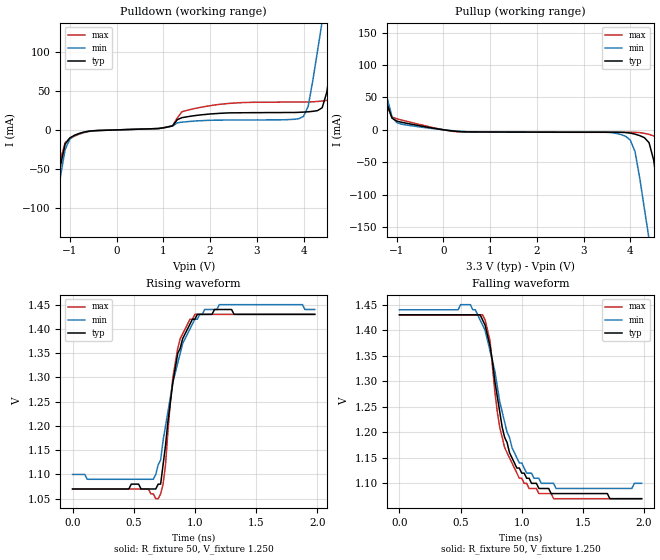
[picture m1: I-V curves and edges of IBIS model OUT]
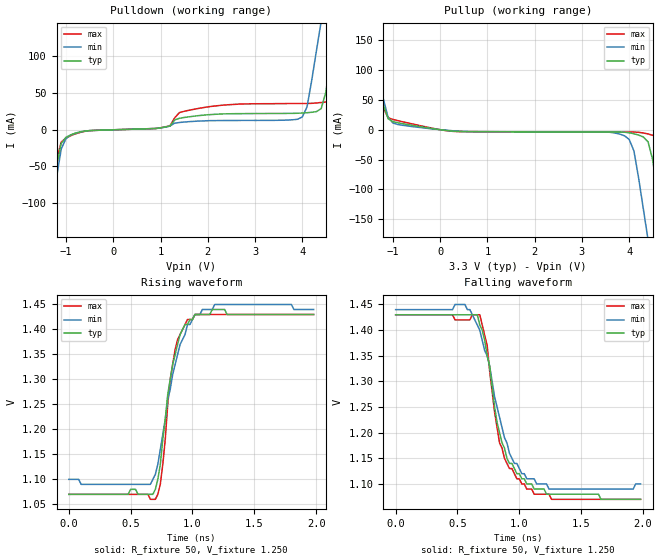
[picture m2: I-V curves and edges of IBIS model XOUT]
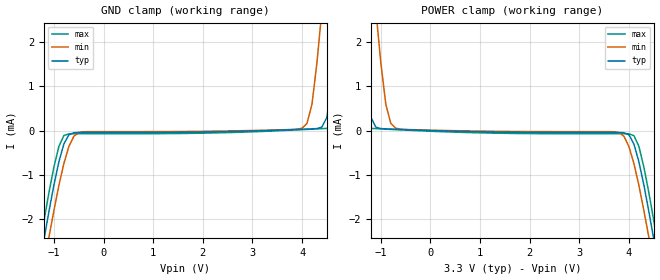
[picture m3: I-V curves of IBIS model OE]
| IBIS File sg5032van_33v.ibs
[IBIS Ver] 3.2
[File name] sg5032van_33v.ibs
[File Rev] 1
[Date] May 1 2013
[Source]
[Disclaimer]
Seiko Epson Corporation makes no warranty with respect to the information
contained herein.
[Copyright]
Copyright(C) 2013 Seiko Epson Corporation. All rights reserved.
| Component SG5032VAN 3.3V
[Component] sg5032van_33v
[Manufacturer] Seiko Epson Corporation
[Package]
R_pkg 0.046 NA NA
L_pkg 0.61n NA NA
C_pkg 0.95p NA NA
[Pin] signal_name model_name R_pin L_pin C_pin
1 OE OE
2 GND GND
3 GND GND
4 OUT OUT 0.046 0.61n 0.95p
5 XOUT XOUT 0.046 0.61n 0.95p
6 VCC POWER
[Diff Pin] inv_pin vdiff tdelay_typ
4 5 0 0
| Models and submodels in the file (3): OUT (Output), XOUT (Output), OE (Input)
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[Model] OUT
Model_type Output
Enable Active-High
Polarity Non-Inverting
Vref=1.250
Vmeas=1.250
Rref=50
Cref=0
C_comp 0.12p 0.12p 0.12p
[Temperature Range] 25 105 -40
[Voltage Range] 3.3 2.97 3.63
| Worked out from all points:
|   slope of the pulldown table from 0 to 0.495 V, typ, clamps not added: 507 ohm
|   slope of the pullup table from 0 to 0.495 V, typ, clamps not added: 153 ohm
|   falling waveform, R_fixture 50, V_fixture 1.250: 20-80 % time 188ps typ, 196ps min, 167ps max; typ from 1.43 V to 1.07 V
|   rising waveform, R_fixture 50, V_fixture 1.250: 20-80 % time 125ps typ, 165ps min, 92.4ps max; typ from 1.07 V to 1.43 V
[Pullup]
-3.3V     961mA      849mA      1.08A
-1.5V     170mA      162mA      181mA
-1.2V     39mA       48.2mA     34.7mA
-900mV    11.8mA     8.83mA     15.3mA
3.9V      -4.13mA    -10mA      -3.85mA
4.1V      -6.66mA    -33.8mA    -3.9mA
4.4V      -19.9mA    -169mA     -7.09mA
4.6V      -99.3mA    -264mA     -12.4mA
4.7V      -153mA     -312mA     -16.5mA
4.8V      -207mA     -360mA     -30.1mA
5.1V      -369mA     -503mA     -198mA
6.6V      -1.18A     -1.22A     -1.1A
[Pulldown]
-3.3V     -1.19A     -1.07A     -1.31A
-1.4V     -152mA     -155mA     -154mA
-1.2V     -45.9mA    -59.6mA    -38.1mA
-1.1V     -18.2mA    -25.2mA    -16.5mA
-900mV    -6.98mA    -7.24mA    -8.05mA
3.9V      22.4mA     14.3mA     35.6mA
4.1V      23.1mA     30mA       35.7mA
4.4V      28.3mA     139mA      36.9mA
4.7V      135mA      253mA      39.9mA
4.8V      179mA      291mA      46.7mA
5V        266mA      366mA      133mA
6.6V      969mA      975mA      937mA
[Falling Waveform]
R_fixture=50
V_fixture=1.250
V_fixture_min=1.271
V_fixture_max=1.238
0s        1.43V      1.44V      1.43V
580ps     1.43V      1.45V      1.43V
680ps     1.42V      1.41V      1.43V
740ps     1.37V      1.36V      1.38V
800ps     1.27V      1.29V      1.24V
860ps     1.19V      1.22V      1.17V
960ps     1.13V      1.15V      1.12V
1.06ns    1.11V      1.12V      1.09V
1.28ns    1.08V      1.09V      1.07V
1.98ns    1.07V      1.1V       1.07V
[Rising Waveform]
R_fixture=50
V_fixture=1.250
V_fixture_min=1.271
V_fixture_max=1.238
0s        1.07V      1.1V       1.07V
660ps     1.07V      1.09V      1.06V
700ps     1.08V      1.12V      1.05V
720ps     1.08V      1.13V      1.06V
740ps     1.12V      1.17V      1.08V
820ps     1.29V      1.29V      1.3V
860ps     1.35V      1.33V      1.36V
1ns       1.42V      1.42V      1.43V
1.2ns     1.44V      1.45V      1.43V
1.98ns    1.43V      1.44V      1.43V
[Ramp]
R_load=50
dV/dt_r 2.133E-1/1.209E-10 2.089E-1/1.701E-10 2.153E-1/9.119E-11
dV/dt_f 2.130E-1/1.860E-10 2.090E-1/2.110E-10 2.147E-1/1.643E-10
|[End OUT
[Model] XOUT
Model_type Output
Enable Active-High
Polarity Inverting
Vref=1.250
Vmeas=1.250
Rref=50
Cref=0
C_comp 0.12p 0.12p 0.12p
[Temperature Range] 25 105 -40
[Voltage Range] 3.3 2.97 3.63
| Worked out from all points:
|   slope of the pulldown table from 0 to 0.495 V, typ, clamps not added: 506 ohm
|   slope of the pullup table from 0 to 0.495 V, typ, clamps not added: 153 ohm
|   falling waveform, R_fixture 50, V_fixture 1.250: 20-80 % time 181ps typ, 204ps min, 151ps max; typ from 1.43 V to 1.07 V
|   rising waveform, R_fixture 50, V_fixture 1.250: 20-80 % time 123ps typ, 159ps min, 93.9ps max; typ from 1.07 V to 1.43 V
[Pullup]
-3.3V     1.03A      904mA      1.18A
-1.5V     183mA      173mA      197mA
-1.2V     41.5mA     51.3mA     36.6mA
-900mV    11.8mA     8.85mA     15.4mA
3.9V      -4.13mA    -10.1mA    -3.85mA
4.1V      -6.68mA    -35.4mA    -3.9mA
4.4V      -20.3mA    -185mA     -7.11mA
4.6V      -110mA     -289mA     -12.4mA
4.7V      -169mA     -341mA     -16.7mA
4.8V      -229mA     -393mA     -31.5mA
5.1V      -408mA     -549mA     -221mA
6.6V      -1.3A      -1.33A     -1.24A
[Pulldown]
-3.3V     -1.32A     -1.17A     -1.48A
-1.4V     -168mA     -170mA     -172mA
-1.2V     -49.6mA    -64.8mA    -40.9mA
-1.1V     -18.6mA    -26.1mA    -16.8mA
-900mV    -7.02mA    -7.27mA    -8.11mA
3.9V      22.5mA     14.3mA     35.7mA
4.1V      23.2mA     31.1mA     35.8mA
4.4V      28.8mA     148mA      37.1mA
4.7V      145mA      269mA      40.2mA
4.8V      192mA      309mA      48.2mA
5V        286mA      390mA      145mA
6.6V      1.04A      1.04A      1.02A
[Falling Waveform]
R_fixture=50
V_fixture=1.250
V_fixture_min=1.271
V_fixture_max=1.238
0s        1.43V      1.44V      1.43V
560ps     1.43V      1.45V      1.42V
660ps     1.43V      1.41V      1.43V
680ps     1.41V      1.4V       1.43V
740ps     1.35V      1.35V      1.37V
840ps     1.2V       1.23V      1.18V
920ps     1.14V      1.16V      1.13V
1.06ns    1.1V       1.11V      1.09V
1.24ns    1.08V      1.09V      1.08V
1.98ns    1.07V      1.1V       1.07V
[Rising Waveform]
R_fixture=50
V_fixture=1.250
V_fixture_min=1.271
V_fixture_max=1.238
0s        1.07V      1.1V       1.07V
660ps     1.07V      1.09V      1.06V
700ps     1.08V      1.11V      1.06V
740ps     1.13V      1.16V      1.09V
780ps     1.22V      1.22V      1.18V
800ps     1.27V      1.26V      1.25V
860ps     1.35V      1.33V      1.36V
960ps     1.41V      1.41V      1.42V
1.18ns    1.44V      1.45V      1.43V
1.98ns    1.43V      1.44V      1.43V
[Ramp]
R_load=50
dV/dt_r 2.132E-1/1.167E-10 2.089E-1/1.633E-10 2.151E-1/9.226E-11
dV/dt_f 2.129E-1/1.808E-10 2.090E-1/2.120E-10 2.145E-1/1.630E-10
|[End XOUT
[Model] OE
Model_type Input
Vinh=2.31
Vinl=0.99
C_comp 3p 3p 3p
[Temperature Range] 25 105 -40
[Voltage Range] 3.3 2.97 3.63
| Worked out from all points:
|   GND clamp passes 1 mA (typ) near -0.96 V on its own axis
|   POWER clamp passes 1 mA (typ) near -1.29 V on its own axis
[GND Clamp]
-3.3V     -17.6mA    -18mA      -17.3mA
-1.2V     -2.46mA    -3.05mA    -2.04mA
-900mV    -706uA     -1.24mA    -357uA
-700mV    -97.5uA    -364uA     -75.2uA
4V        28.3uA     52.1uA     20.1uA
4.2V      37.3uA     598uA      31.3uA
4.4V      76.9uA     2.73mA     42.7uA
4.5V      301uA      3.93mA     48.4uA
4.7V      2.34mA     6.32mA     64.4uA
4.8V      3.63mA     7.51mA     145uA
5.1V      7.52mA     11.1mA     3.36mA
6.6V      27mA       29.1mA     24.2mA
[POWER Clamp]
-3.3V     27mA       29.1mA     24.2mA
-1.8V     7.52mA     11.1mA     3.36mA
-1.5V     3.63mA     7.51mA     145uA
-1.4V     2.34mA     6.32mA     64.4uA
-1.2V     301uA      3.93mA     48.4uA
-1.1V     76.9uA     2.73mA     42.7uA
-900mV    37.3uA     598uA      31.3uA
-700mV    28.3uA     52.1uA     20.1uA
4V        -97.5uA    -364uA     -75.2uA
4.2V      -706uA     -1.24mA    -357uA
4.5V      -2.46mA    -3.05mA    -2.04mA
6.6V      -17.6mA    -18mA      -17.3mA
